(* Logix 5000 AddOnInstructionDefinition export Banner_S15C_UI_Param_v2; software revision 32.00 *)

TYPE Banner_IOL_Port_v2 :   // UDT that has all of the data items necessary to communicate with a specific Port on a IO-Link Master
STRUCT
   Port_Controlled : INT;   // Each bit represents a port on an IO-Link Master. Set to 1 to tell AOI to control that port.
   Port_Activate : INT;   // Each bit represents a port on an IO-Link Master. When ON that port will process any commands in queue.
   Port_Read : INT;   // Each bit represents a port on an IO-Link Master. Used to determine when device AOI has requested a Read command.
   Port_Write : INT;   // Each bit represents a port on an IO-Link Master. Used to determine when device AOI has requested a Write command.
   Port_RW_Complete : INT;   // Each bit represents a port on an IO-Link Master. Tells device AOI that Read or Write request has been completed.
   Port_Device_Read : INT;
   Data_Transfer : SINT[70];   // Array to transfer data from IO-Master to device AOIs.
END_STRUCT
END_TYPE

TYPE Banner_S15C_UI_RD_v2 :   // All of the read parameters for a S15C-IU unit.
STRUCT
   Master_Cycle_Time : INT;
   Min_Cycle_Time : INT;
   M_Sequence_Capability : INT;
   IO_Link_Version_ID : INT;
   Process_Data_Input_Length : INT;
   Process_Data_Output_Length : INT;
   Combined_Vendor_ID : DINT;   // IO-Link Vendor ID
   Vendor_ID1 : INT;
   Vendor_ID2 : INT;
   Combined_Device_ID : DINT;   // IO-Link Device ID
   Device_ID1 : INT;
   Device_ID2 : INT;
   Device_ID3 : INT;
   Serial_Number : STRING;
   Product_Name : STRING;
   All_Time_Run_Time : DINT;   // Current All Time Run Timer.
   Model_Type : SINT;   // 0 = Voltage, 1 = Current
   MDC_Lower_Limit : DINT;
   MDC_Upper_Limit : DINT;
   MDC_Unit : DINT;   // 1209 = A, 1240 = V
   MDC_Scale : DINT;   // 260 = microAmps, 253 = microVolts
END_STRUCT
END_TYPE

TYPE Banner_S15C_UI_v2 :   // All of the parameters for a S15C.
STRUCT
   Initial_Global_Read : BOOL;   // Determines if all of the IO-Link data has been read into the PLC yet
   Command : INT;   // Value placed in here will activate a read or write to a specifc IO-Link Index
   Read_Data : Banner_S15C_UI_RD_v2;   // Read Only Data
   Write_Data : Banner_S15C_UI_WD_v2;   // Write Data
   Archive : Banner_S15C_UI_WD_v2;   // Archive Data
   Reset : BOOL;   // Resets AOI. This will force a complete parameter read of the sensor.
END_STRUCT
END_TYPE

TYPE Banner_S15C_UI_WD_v2 :   // UDT that stores the Write Data for a S15C-IU unit.
STRUCT
   System_Command : INT;   // See IODD file for list of commands that can be activated via the System Command interface
   Parameter_Access_Lock : SINT;   // Write access to all parameters is prohibited while value is 1. Only this parameter can be adjusted when value is 1.
   Data_Storage_Lock : SINT;   // Automatic data storage is disabled when this value is equal to 1. Read access is not affected.
   Local_Parameterization_Lock : SINT;   // Parameterization via local control elements on device is disabled.
   Local_User_Interface_Lock : SINT;   // Operation of local user interface is disabled.
   Setpoint_SP1 : DINT;
   Setpoint_SP2 : DINT;
   Switchpoint_Logic : INT;   // 0 = Light Operate, 1 = Dark Operate
   BDC_Mode : INT;   // 2 = Window Mode.
   Hysteresis : DINT;   // Hysteresis value for the switchpoint.
   Resetable_Run_Time : DINT;   // Current Resetable Run Timer.
   PDI_Configuration : INT;   // 0 = Analog Value, 1 = Digital Measuring Sensor
   IOL_Filter_Time : DINT;   // Time to average IOL Process Data management between updates.
   All_Time_Run_Time_Event_Time : DINT;   // Time before an Event is generated. 0 = disable all-time event.
   Resetable_Run_Time_Event_Time : DINT;   // Time before an Event is generated. 0 = disable run time event.
END_STRUCT
END_TYPE

ADD_ON_INSTRUCTION Banner_S15C_UI_Param_v2   (* revision 2.1, vendor Banner Engineering *)
// AOI to read and write parameter data to an IO-Link S15C-I or S15C-U.
VAR_IN_OUT
   S15C : Banner_S15C_UI_v2; {required}
   Port_Data : Banner_IOL_Port_v2; {required}
END_VAR
VAR_INPUT
   Port : DINT; {required}
END_VAR
VAR
   Local_Control : DINT; {access None}
   Global_Read_Command_Value : INT; {access None}
   Global_Write_Command_Value : INT; {access None}
   Error_Generated : BOOL; {access None}
   Command_Being_Processed : BOOL; {access None}
   Index_Write_Inprocess : INT; {access None}
   Index_Write_Control : INT; {access None}
   Update_Archive : BOOL; {access None}
   Inprocess_Index : DINT; {access None}
END_VAR

ROUTINE Logic   (* ladder *)
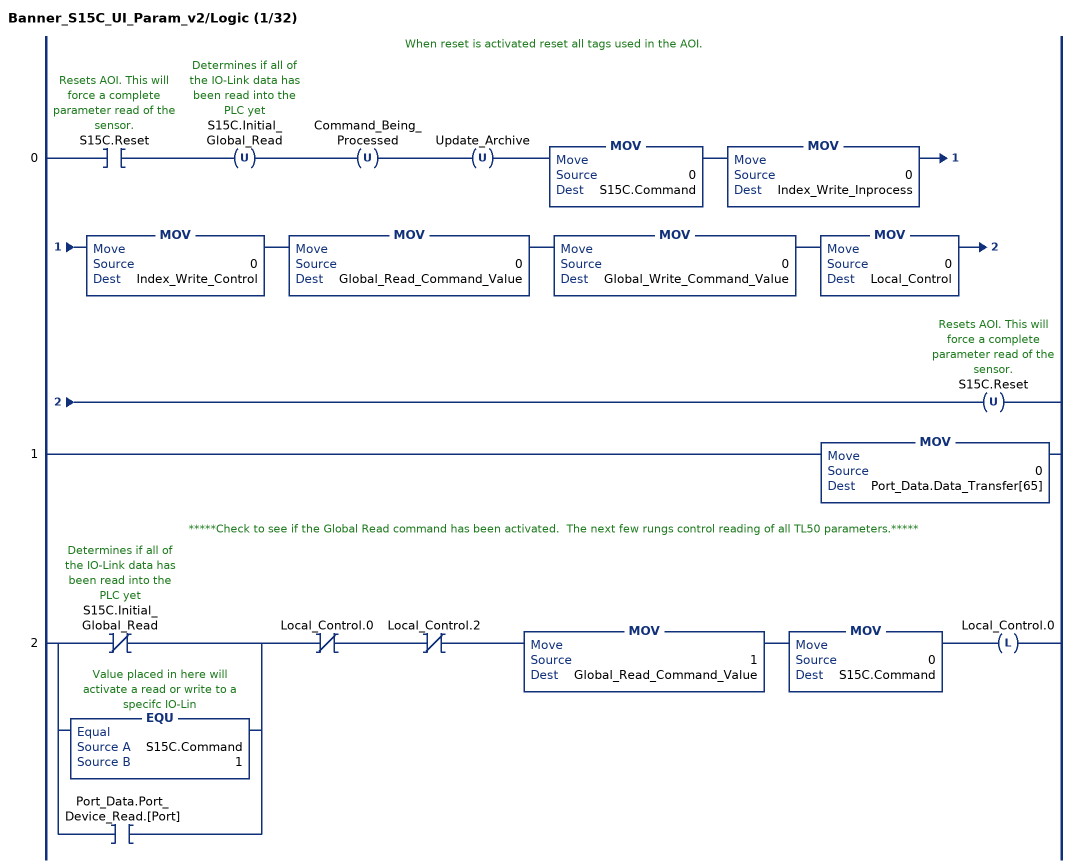
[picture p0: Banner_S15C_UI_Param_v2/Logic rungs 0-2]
   // When reset is activated reset all tags used in the AOI.
   0: XIC(S15C.Reset)OTU(S15C.Initial_Global_Read)OTU(Command_Being_Processed)OTU(Update_Archive)MOV(0,S15C.Command)MOV(0,Index_Write_Inprocess)MOV(0,Index_Write_Control)MOV(0,Global_Read_Command_Value)MOV(0,Global_Write_Command_Value)MOV(0,Local_Control)OTU(S15C.Reset);
   1: MOV(0,Port_Data.Data_Transfer[65]);
   // *****Check to see if the Global Read command has been activated.  The next few rungs control reading of all TL50 parameters.*****
   2: [XIO(S15C.Initial_Global_Read) ,EQU(S15C.Command,1) ,XIC(Port_Data.Port_Device_Read.[Port]) ]XIO(Local_Control.0)XIO(Local_Control.2)MOV(1,Global_Read_Command_Value)MOV(0,S15C.Command)OTL(Local_Control.0);
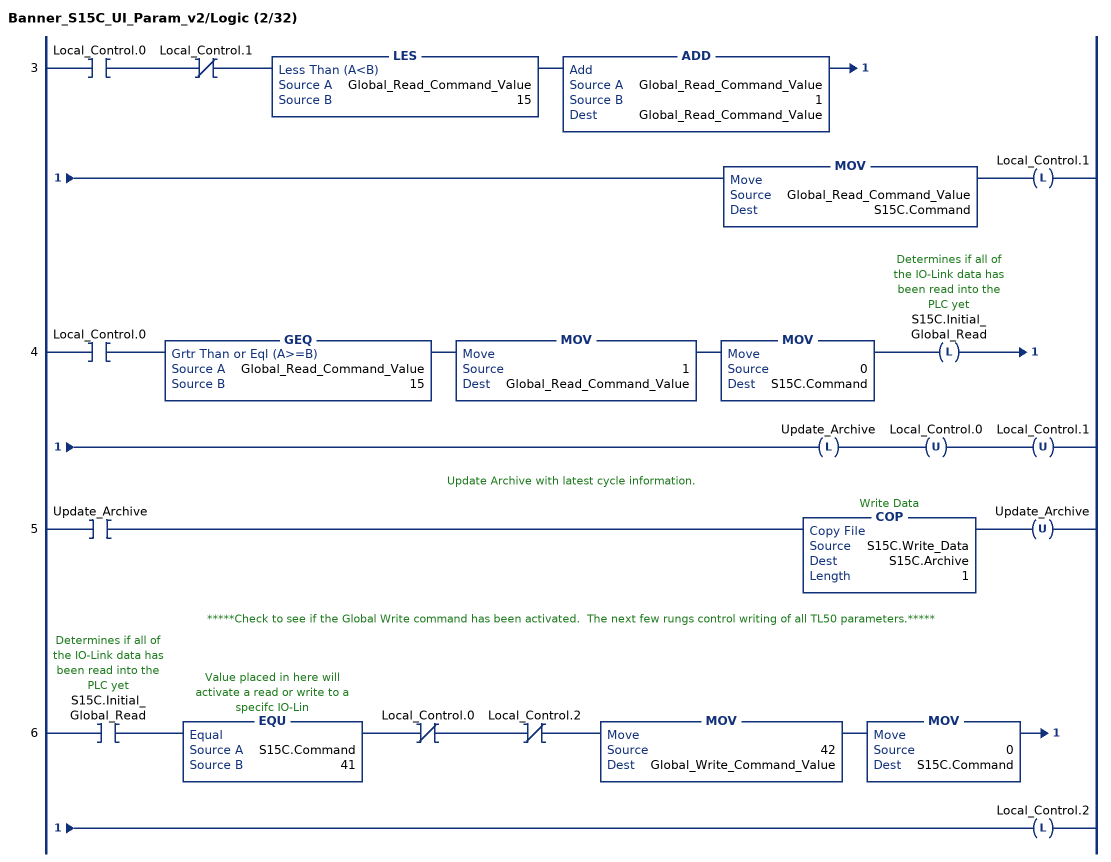
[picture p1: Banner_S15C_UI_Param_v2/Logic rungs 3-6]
   3: XIC(Local_Control.0)XIO(Local_Control.1)LES(Global_Read_Command_Value,15)ADD(Global_Read_Command_Value,1,Global_Read_Command_Value)MOV(Global_Read_Command_Value,S15C.Command)OTL(Local_Control.1);
   4: XIC(Local_Control.0)GEQ(Global_Read_Command_Value,15)MOV(1,Global_Read_Command_Value)MOV(0,S15C.Command)OTL(S15C.Initial_Global_Read)OTL(Update_Archive)OTU(Local_Control.0)OTU(Local_Control.1);
   // Update Archive with latest cycle information.
   5: XIC(Update_Archive)COP(S15C.Write_Data,S15C.Archive,1)OTU(Update_Archive);
   // *****Check to see if the Global Write command has been activated.  The next few rungs control writing of all TL50 parameters.*****
   6: XIC(S15C.Initial_Global_Read)EQU(S15C.Command,41)XIO(Local_Control.0)XIO(Local_Control.2)MOV(42,Global_Write_Command_Value)MOV(0,S15C.Command)OTL(Local_Control.2);
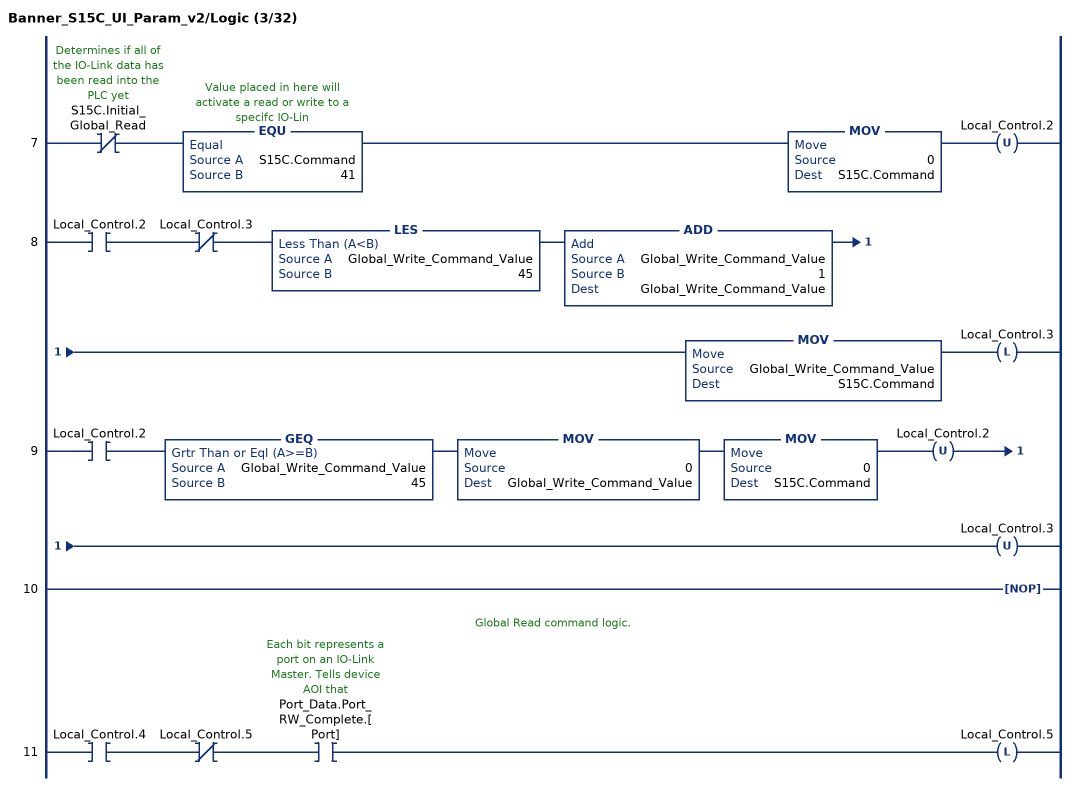
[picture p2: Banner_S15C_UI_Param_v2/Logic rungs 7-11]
   7: XIO(S15C.Initial_Global_Read)EQU(S15C.Command,41)MOV(0,S15C.Command)OTU(Local_Control.2);
   8: XIC(Local_Control.2)XIO(Local_Control.3)LES(Global_Write_Command_Value,45)ADD(Global_Write_Command_Value,1,Global_Write_Command_Value)MOV(Global_Write_Command_Value,S15C.Command)OTL(Local_Control.3);
   9: XIC(Local_Control.2)GEQ(Global_Write_Command_Value,45)MOV(0,Global_Write_Command_Value)MOV(0,S15C.Command)OTU(Local_Control.2)OTU(Local_Control.3);
   10: NOP();
   // Global Read command logic.
   11: XIC(Local_Control.4)XIO(Local_Control.5)XIC(Port_Data.Port_RW_Complete.[Port])OTL(Local_Control.5);
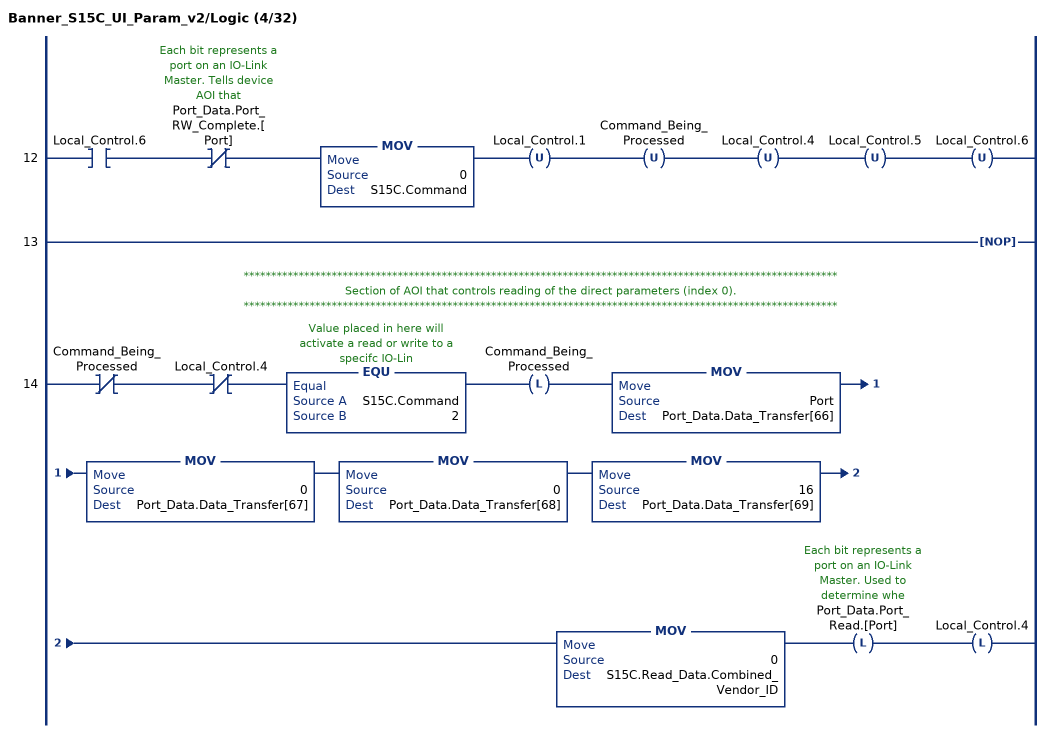
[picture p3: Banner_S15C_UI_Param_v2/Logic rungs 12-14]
   12: XIC(Local_Control.6)XIO(Port_Data.Port_RW_Complete.[Port])MOV(0,S15C.Command)OTU(Local_Control.1)OTU(Command_Being_Processed)OTU(Local_Control.4)OTU(Local_Control.5)OTU(Local_Control.6);
   13: NOP();
   // ************************************************************************************************************
   // Section of AOI that controls reading of the direct parameters (index 0).
   // ************************************************************************************************************
   14: XIO(Command_Being_Processed)XIO(Local_Control.4)EQU(S15C.Command,2)OTL(Command_Being_Processed)MOV(Port,Port_Data.Data_Transfer[66])MOV(0,Port_Data.Data_Transfer[67])MOV(0,Port_Data.Data_Transfer[68])MOV(16,Port_Data.Data_Transfer[69])MOV(0,S15C.Read_Data.Combined_Vendor_ID)OTL(Port_Data.Port_Read.[Port])OTL(Local_Control.4);
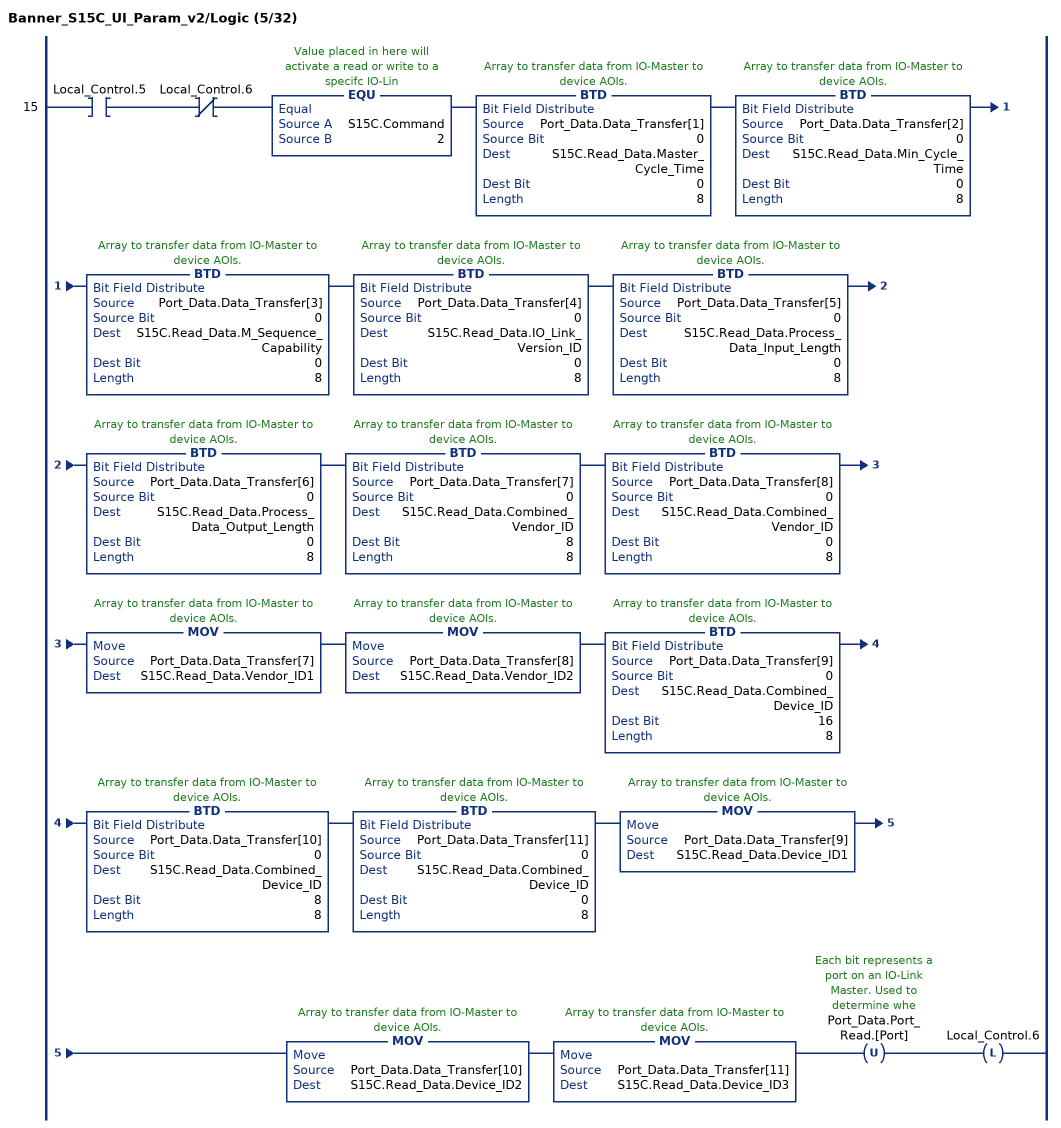
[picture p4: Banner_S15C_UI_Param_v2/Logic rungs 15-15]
   15: XIC(Local_Control.5)XIO(Local_Control.6)EQU(S15C.Command,2)BTD(Port_Data.Data_Transfer[1],0,S15C.Read_Data.Master_Cycle_Time,0,8)BTD(Port_Data.Data_Transfer[2],0,S15C.Read_Data.Min_Cycle_Time,0,8)BTD(Port_Data.Data_Transfer[3],0,S15C.Read_Data.M_Sequence_Capability,0,8)BTD(Port_Data.Data_Transfer[4],0,S15C.Read_Data.IO_Link_Version_ID,0,8)BTD(Port_Data.Data_Transfer[5],0,S15C.Read_Data.Process_Data_Input_Length,0,8)BTD(Port_Data.Data_Transfer[6],0,S15C.Read_Data.Process_Data_Output_Length,0,8)BTD(Port_Data.Data_Transfer[7],0,S15C.Read_Data.Combined_Vendor_ID,8,8)BTD(Port_Data.Data_Transfer[8],0,S15C.Read_Data.Combined_Vendor_ID,0,8)MOV(Port_Data.Data_Transfer[7],S15C.Read_Data.Vendor_ID1)MOV(Port_Data.Data_Transfer[8],S15C.Read_Data.Vendor_ID2)BTD(Port_Data.Data_Transfer[9],0,S15C.Read_Data.Combined_Device_ID,16,8)BTD(Port_Data.Data_Transfer[10],0,S15C.Read_Data.Combined_Device_ID,8,8)BTD(Port_Data.Data_Transfer[11],0,S15C.Read_Data.Combined_Device_ID,0,8)MOV(Port_Data.Data_Transfer[9],S15C.Read_Data.Device_ID1)MOV(Port_Data.Data_Transfer[10],S15C.Read_Data.Device_ID2)MOV(Port_Data.Data_Transfer[11],S15C.Read_Data.Device_ID3)OTU(Port_Data.Port_Read.[Port])OTL(Local_Control.6);
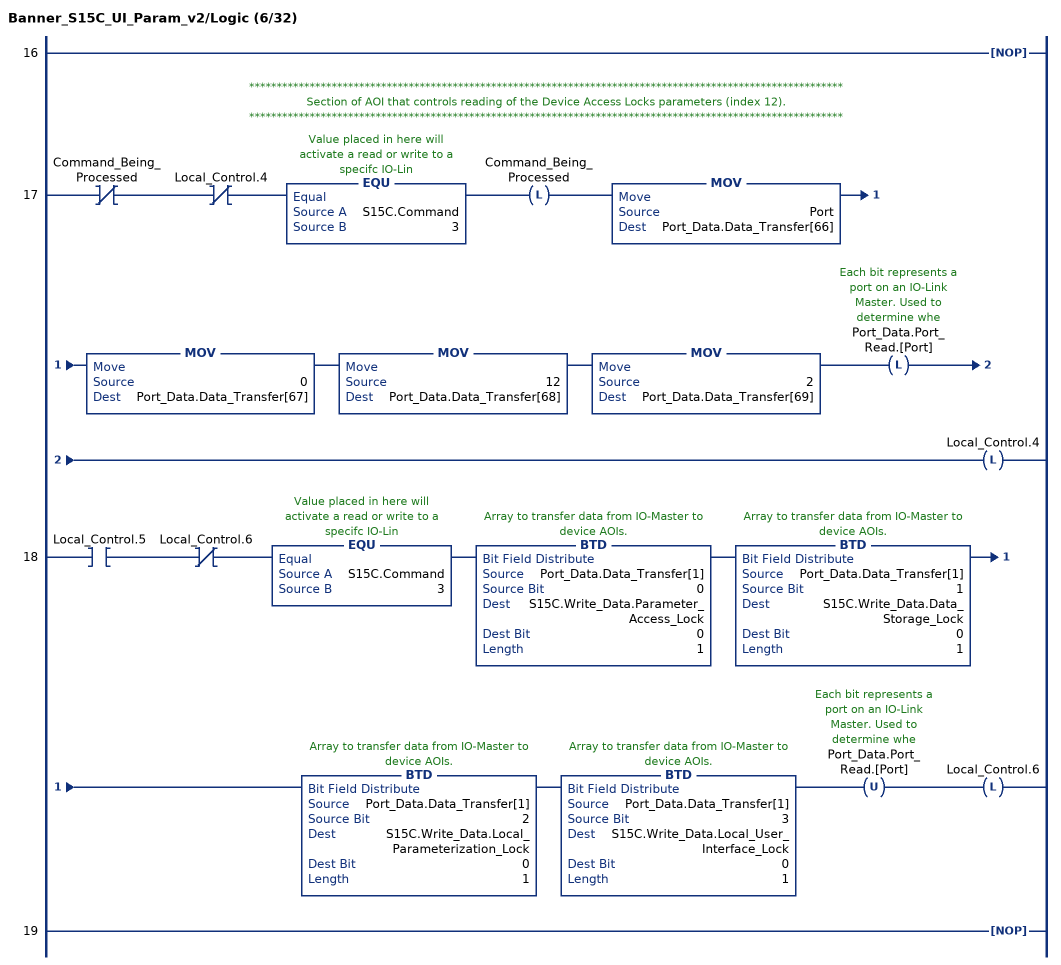
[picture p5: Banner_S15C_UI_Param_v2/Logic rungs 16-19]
   16: NOP();
   // ************************************************************************************************************
   // Section of AOI that controls reading of the Device Access Locks parameters (index 12).
   // ************************************************************************************************************
   17: XIO(Command_Being_Processed)XIO(Local_Control.4)EQU(S15C.Command,3)OTL(Command_Being_Processed)MOV(Port,Port_Data.Data_Transfer[66])MOV(0,Port_Data.Data_Transfer[67])MOV(12,Port_Data.Data_Transfer[68])MOV(2,Port_Data.Data_Transfer[69])OTL(Port_Data.Port_Read.[Port])OTL(Local_Control.4);
   18: XIC(Local_Control.5)XIO(Local_Control.6)EQU(S15C.Command,3)BTD(Port_Data.Data_Transfer[1],0,S15C.Write_Data.Parameter_Access_Lock,0,1)BTD(Port_Data.Data_Transfer[1],1,S15C.Write_Data.Data_Storage_Lock,0,1)BTD(Port_Data.Data_Transfer[1],2,S15C.Write_Data.Local_Parameterization_Lock,0,1)BTD(Port_Data.Data_Transfer[1],3,S15C.Write_Data.Local_User_Interface_Lock,0,1)OTU(Port_Data.Port_Read.[Port])OTL(Local_Control.6);
   19: NOP();
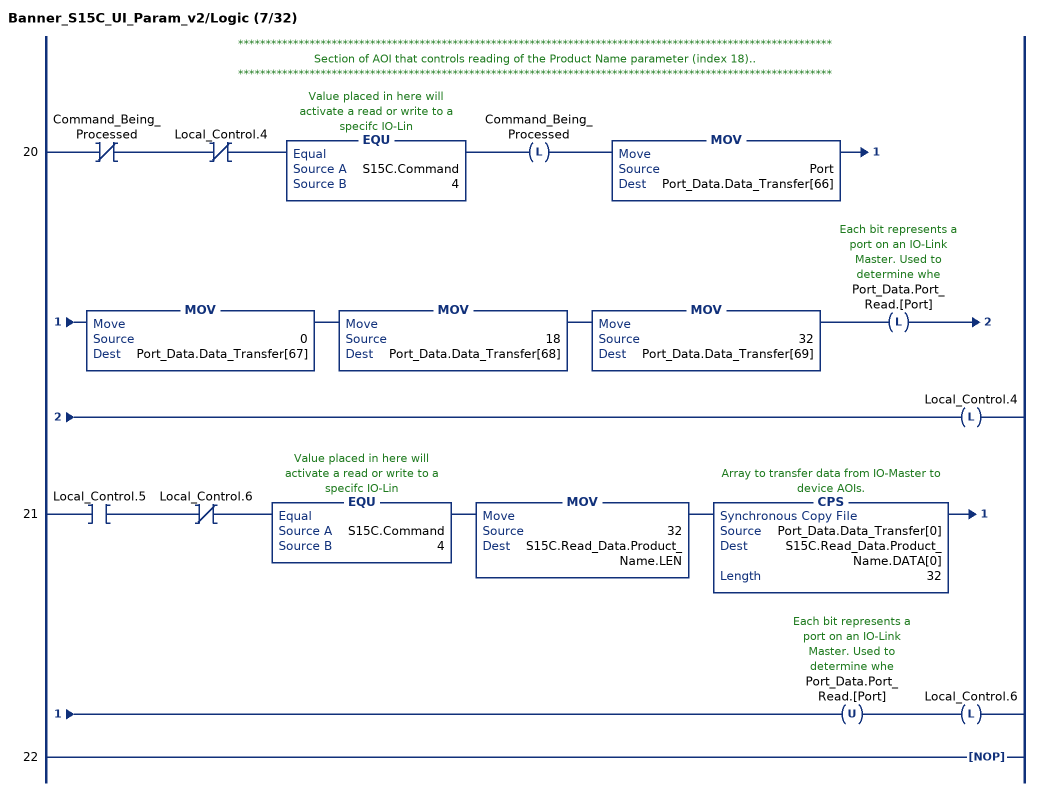
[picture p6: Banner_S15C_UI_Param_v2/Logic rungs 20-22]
   // ************************************************************************************************************
   // Section of AOI that controls reading of the Product Name parameter (index 18)..
   // ************************************************************************************************************
   20: XIO(Command_Being_Processed)XIO(Local_Control.4)EQU(S15C.Command,4)OTL(Command_Being_Processed)MOV(Port,Port_Data.Data_Transfer[66])MOV(0,Port_Data.Data_Transfer[67])MOV(18,Port_Data.Data_Transfer[68])MOV(32,Port_Data.Data_Transfer[69])OTL(Port_Data.Port_Read.[Port])OTL(Local_Control.4);
   21: XIC(Local_Control.5)XIO(Local_Control.6)EQU(S15C.Command,4)MOV(32,S15C.Read_Data.Product_Name.LEN)CPS(Port_Data.Data_Transfer[0],S15C.Read_Data.Product_Name.DATA[0],32)OTU(Port_Data.Port_Read.[Port])OTL(Local_Control.6);
   22: NOP();
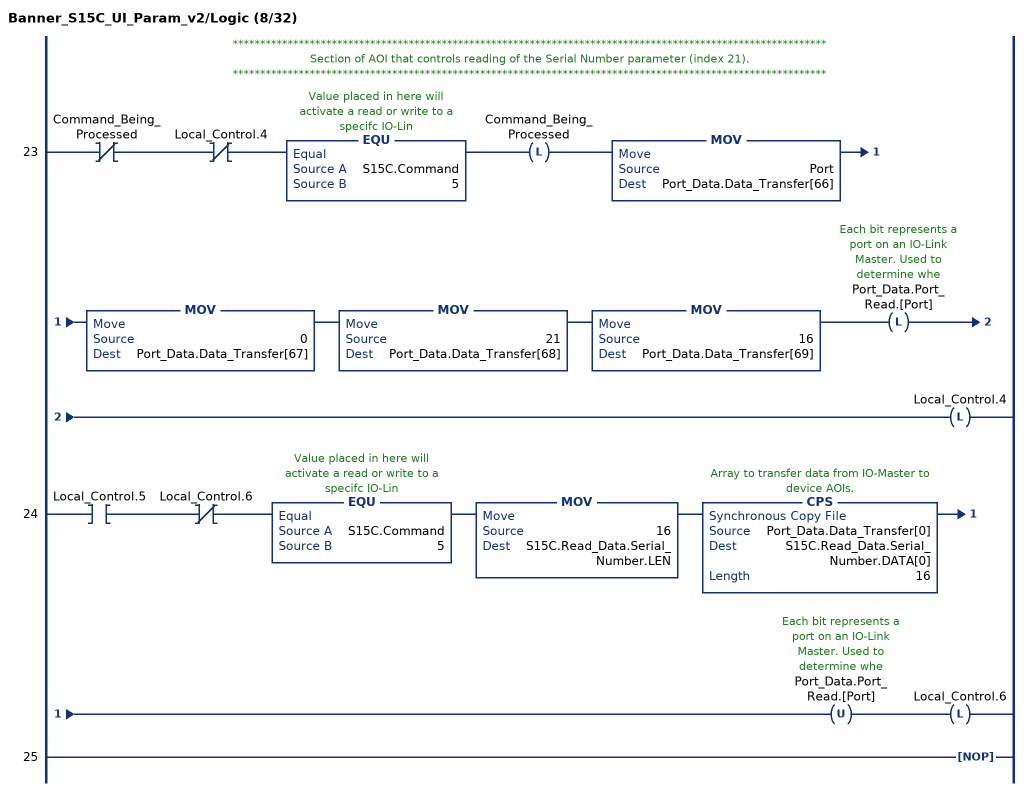
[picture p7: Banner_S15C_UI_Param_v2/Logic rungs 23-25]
   // ************************************************************************************************************
   // Section of AOI that controls reading of the Serial Number parameter (index 21).
   // ************************************************************************************************************
   23: XIO(Command_Being_Processed)XIO(Local_Control.4)EQU(S15C.Command,5)OTL(Command_Being_Processed)MOV(Port,Port_Data.Data_Transfer[66])MOV(0,Port_Data.Data_Transfer[67])MOV(21,Port_Data.Data_Transfer[68])MOV(16,Port_Data.Data_Transfer[69])OTL(Port_Data.Port_Read.[Port])OTL(Local_Control.4);
   24: XIC(Local_Control.5)XIO(Local_Control.6)EQU(S15C.Command,5)MOV(16,S15C.Read_Data.Serial_Number.LEN)CPS(Port_Data.Data_Transfer[0],S15C.Read_Data.Serial_Number.DATA[0],16)OTU(Port_Data.Port_Read.[Port])OTL(Local_Control.6);
   25: NOP();
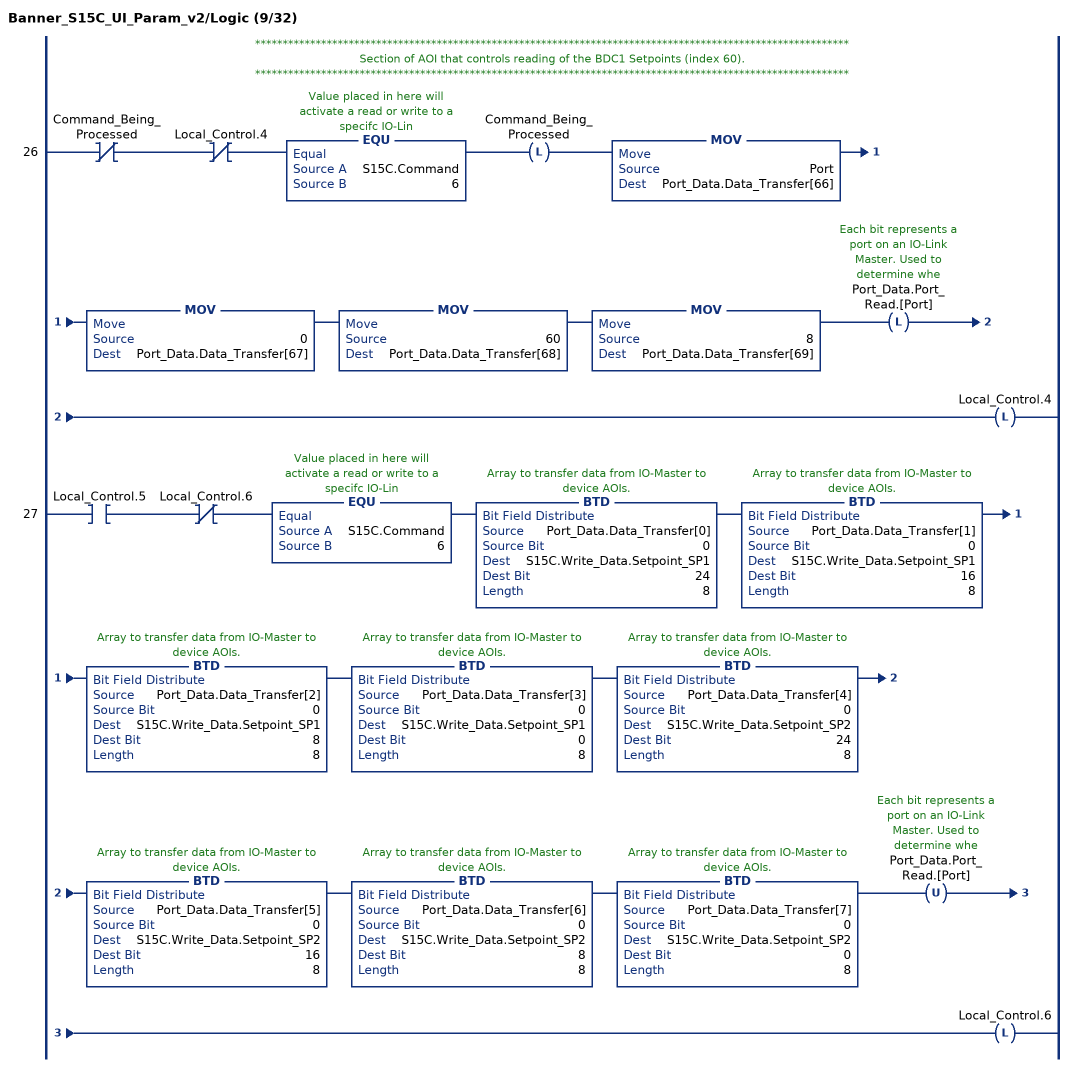
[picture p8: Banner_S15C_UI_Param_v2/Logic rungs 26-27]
   // ************************************************************************************************************
   // Section of AOI that controls reading of the BDC1 Setpoints (index 60).
   // ************************************************************************************************************
   26: XIO(Command_Being_Processed)XIO(Local_Control.4)EQU(S15C.Command,6)OTL(Command_Being_Processed)MOV(Port,Port_Data.Data_Transfer[66])MOV(0,Port_Data.Data_Transfer[67])MOV(60,Port_Data.Data_Transfer[68])MOV(8,Port_Data.Data_Transfer[69])OTL(Port_Data.Port_Read.[Port])OTL(Local_Control.4);
   27: XIC(Local_Control.5)XIO(Local_Control.6)EQU(S15C.Command,6)BTD(Port_Data.Data_Transfer[0],0,S15C.Write_Data.Setpoint_SP1,24,8)BTD(Port_Data.Data_Transfer[1],0,S15C.Write_Data.Setpoint_SP1,16,8)BTD(Port_Data.Data_Transfer[2],0,S15C.Write_Data.Setpoint_SP1,8,8)BTD(Port_Data.Data_Transfer[3],0,S15C.Write_Data.Setpoint_SP1,0,8)BTD(Port_Data.Data_Transfer[4],0,S15C.Write_Data.Setpoint_SP2,24,8)BTD(Port_Data.Data_Transfer[5],0,S15C.Write_Data.Setpoint_SP2,16,8)BTD(Port_Data.Data_Transfer[6],0,S15C.Write_Data.Setpoint_SP2,8,8)BTD(Port_Data.Data_Transfer[7],0,S15C.Write_Data.Setpoint_SP2,0,8)OTU(Port_Data.Port_Read.[Port])OTL(Local_Control.6);
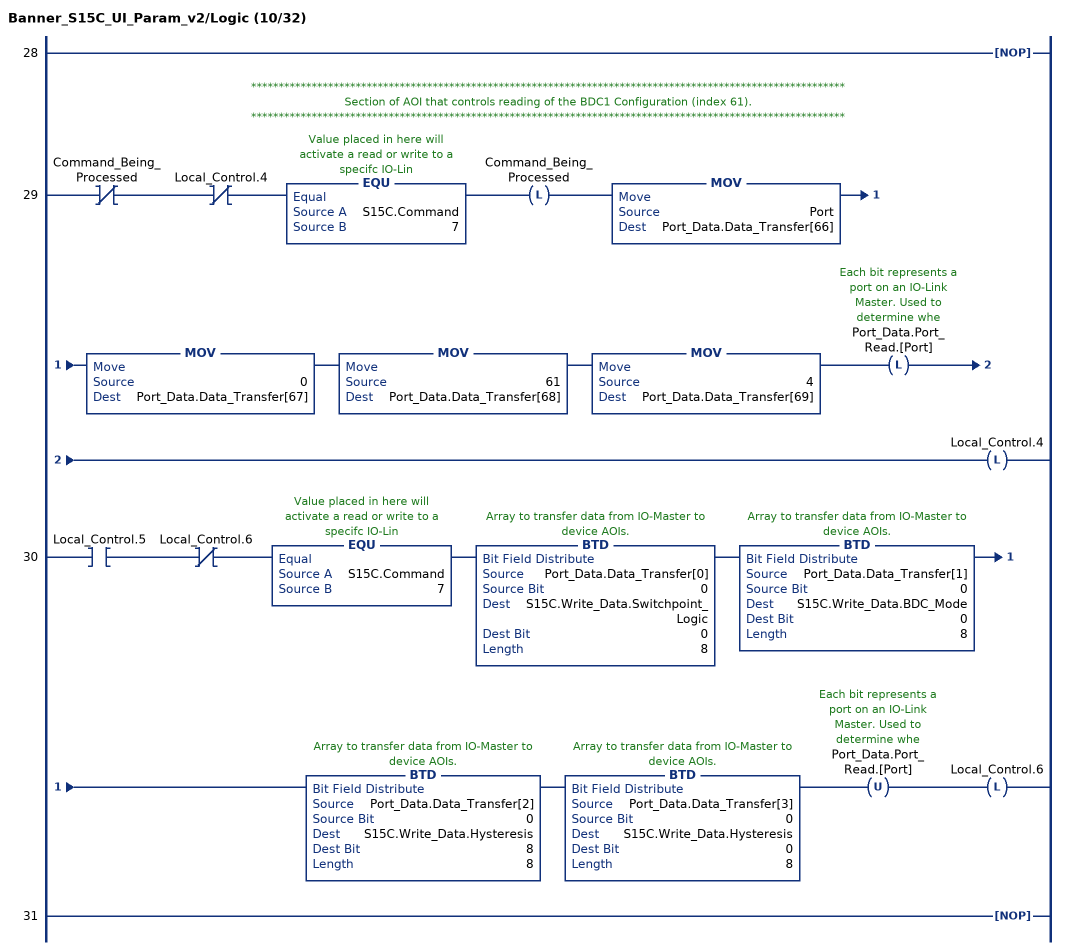
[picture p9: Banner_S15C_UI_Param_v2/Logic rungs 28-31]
   28: NOP();
   // ************************************************************************************************************
   // Section of AOI that controls reading of the BDC1 Configuration (index 61).
   // ************************************************************************************************************
   29: XIO(Command_Being_Processed)XIO(Local_Control.4)EQU(S15C.Command,7)OTL(Command_Being_Processed)MOV(Port,Port_Data.Data_Transfer[66])MOV(0,Port_Data.Data_Transfer[67])MOV(61,Port_Data.Data_Transfer[68])MOV(4,Port_Data.Data_Transfer[69])OTL(Port_Data.Port_Read.[Port])OTL(Local_Control.4);
   30: XIC(Local_Control.5)XIO(Local_Control.6)EQU(S15C.Command,7)BTD(Port_Data.Data_Transfer[0],0,S15C.Write_Data.Switchpoint_Logic,0,8)BTD(Port_Data.Data_Transfer[1],0,S15C.Write_Data.BDC_Mode,0,8)BTD(Port_Data.Data_Transfer[2],0,S15C.Write_Data.Hysteresis,8,8)BTD(Port_Data.Data_Transfer[3],0,S15C.Write_Data.Hysteresis,0,8)OTU(Port_Data.Port_Read.[Port])OTL(Local_Control.6);
   31: NOP();
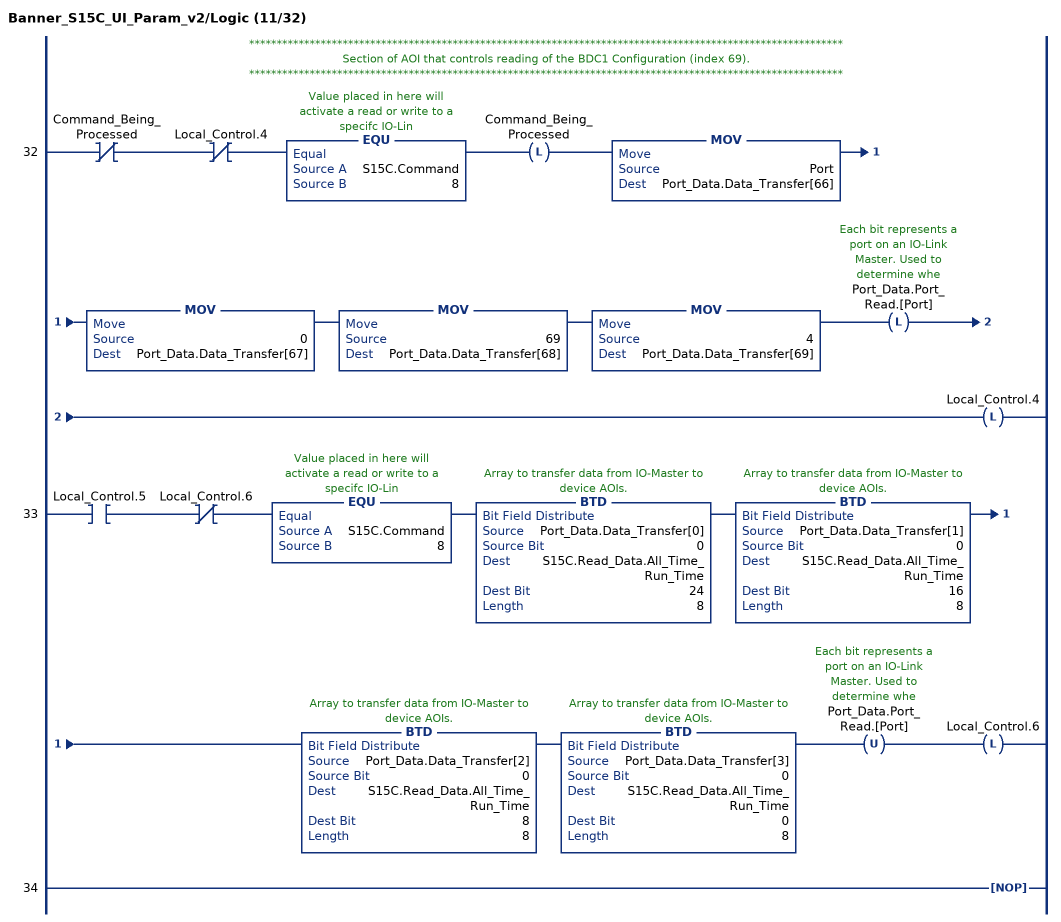
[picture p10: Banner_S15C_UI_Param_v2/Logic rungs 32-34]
   // ************************************************************************************************************
   // Section of AOI that controls reading of the BDC1 Configuration (index 69).
   // ************************************************************************************************************
   32: XIO(Command_Being_Processed)XIO(Local_Control.4)EQU(S15C.Command,8)OTL(Command_Being_Processed)MOV(Port,Port_Data.Data_Transfer[66])MOV(0,Port_Data.Data_Transfer[67])MOV(69,Port_Data.Data_Transfer[68])MOV(4,Port_Data.Data_Transfer[69])OTL(Port_Data.Port_Read.[Port])OTL(Local_Control.4);
   33: XIC(Local_Control.5)XIO(Local_Control.6)EQU(S15C.Command,8)BTD(Port_Data.Data_Transfer[0],0,S15C.Read_Data.All_Time_Run_Time,24,8)BTD(Port_Data.Data_Transfer[1],0,S15C.Read_Data.All_Time_Run_Time,16,8)BTD(Port_Data.Data_Transfer[2],0,S15C.Read_Data.All_Time_Run_Time,8,8)BTD(Port_Data.Data_Transfer[3],0,S15C.Read_Data.All_Time_Run_Time,0,8)OTU(Port_Data.Port_Read.[Port])OTL(Local_Control.6);
   34: NOP();
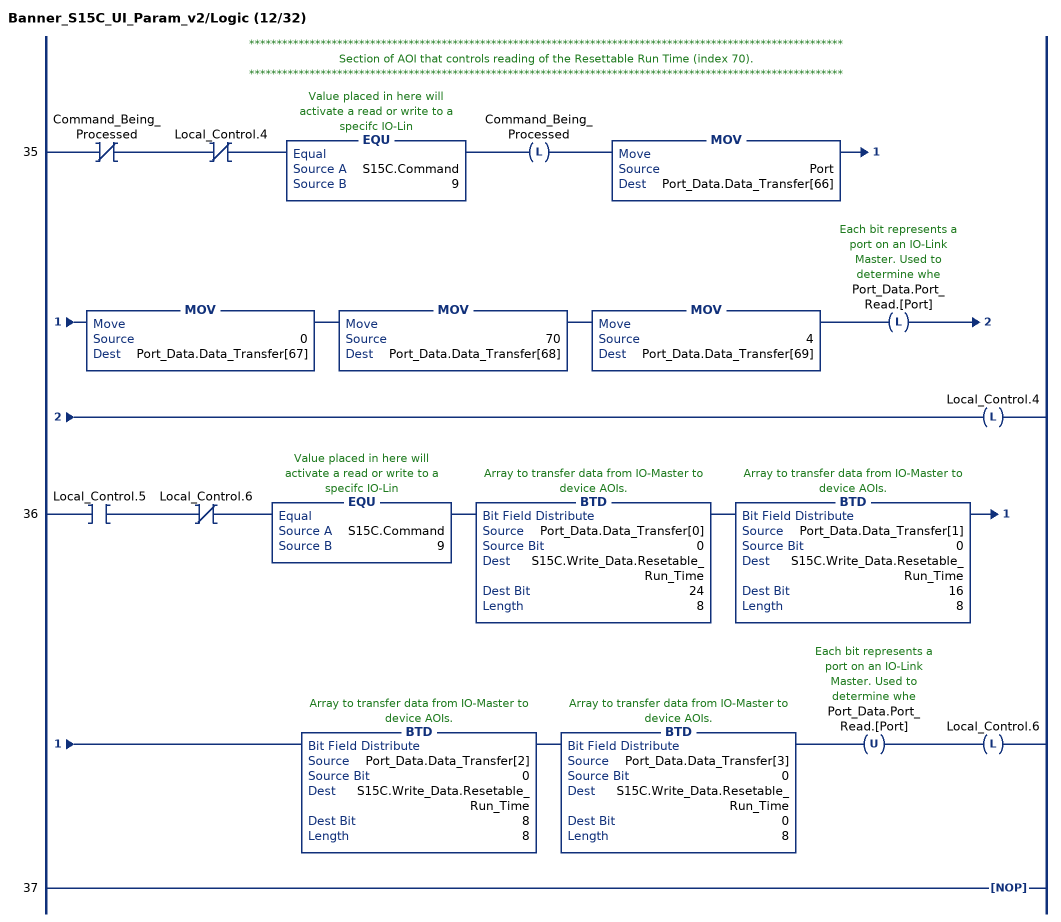
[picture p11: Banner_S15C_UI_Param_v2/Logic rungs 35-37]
   // ************************************************************************************************************
   // Section of AOI that controls reading of the Resettable Run Time (index 70).
   // ************************************************************************************************************
   35: XIO(Command_Being_Processed)XIO(Local_Control.4)EQU(S15C.Command,9)OTL(Command_Being_Processed)MOV(Port,Port_Data.Data_Transfer[66])MOV(0,Port_Data.Data_Transfer[67])MOV(70,Port_Data.Data_Transfer[68])MOV(4,Port_Data.Data_Transfer[69])OTL(Port_Data.Port_Read.[Port])OTL(Local_Control.4);
   36: XIC(Local_Control.5)XIO(Local_Control.6)EQU(S15C.Command,9)BTD(Port_Data.Data_Transfer[0],0,S15C.Write_Data.Resetable_Run_Time,24,8)BTD(Port_Data.Data_Transfer[1],0,S15C.Write_Data.Resetable_Run_Time,16,8)BTD(Port_Data.Data_Transfer[2],0,S15C.Write_Data.Resetable_Run_Time,8,8)BTD(Port_Data.Data_Transfer[3],0,S15C.Write_Data.Resetable_Run_Time,0,8)OTU(Port_Data.Port_Read.[Port])OTL(Local_Control.6);
   37: NOP();
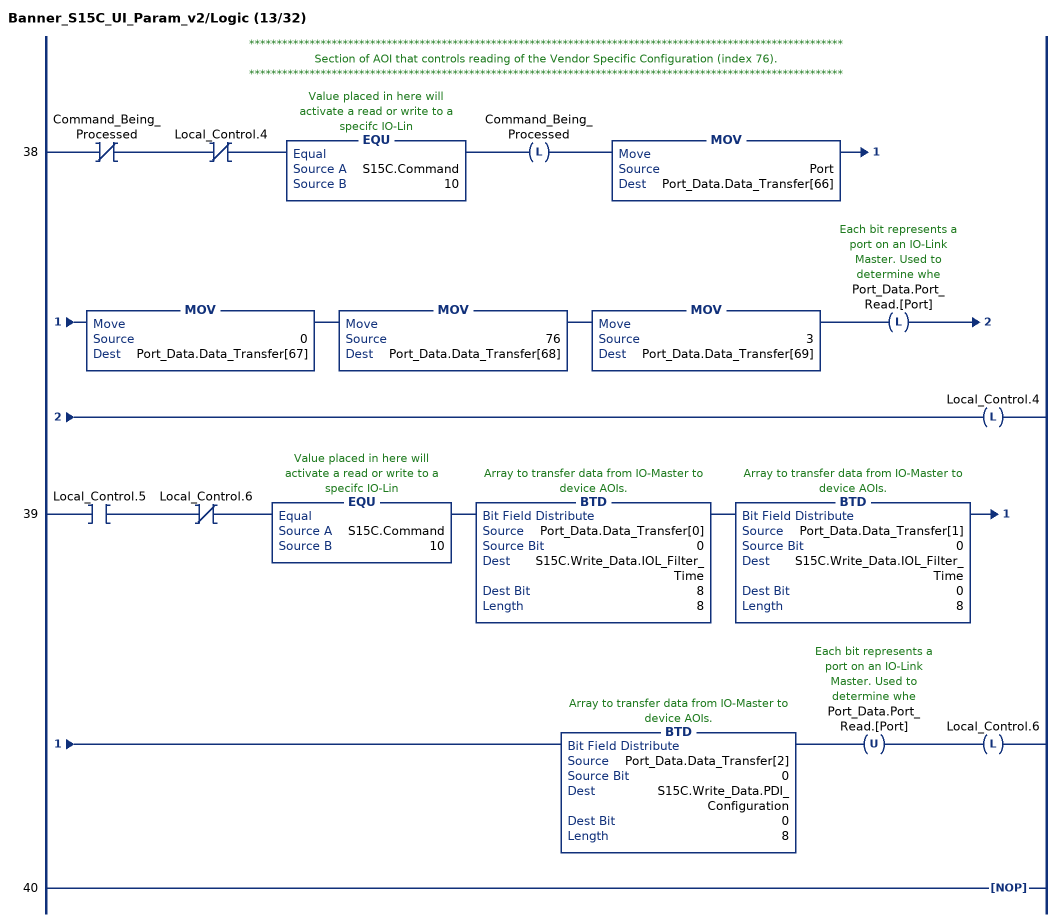
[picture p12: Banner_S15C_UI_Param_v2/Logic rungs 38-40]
   // ************************************************************************************************************
   // Section of AOI that controls reading of the Vendor Specific Configuration (index 76).
   // ************************************************************************************************************
   38: XIO(Command_Being_Processed)XIO(Local_Control.4)EQU(S15C.Command,10)OTL(Command_Being_Processed)MOV(Port,Port_Data.Data_Transfer[66])MOV(0,Port_Data.Data_Transfer[67])MOV(76,Port_Data.Data_Transfer[68])MOV(3,Port_Data.Data_Transfer[69])OTL(Port_Data.Port_Read.[Port])OTL(Local_Control.4);
   39: XIC(Local_Control.5)XIO(Local_Control.6)EQU(S15C.Command,10)BTD(Port_Data.Data_Transfer[0],0,S15C.Write_Data.IOL_Filter_Time,8,8)BTD(Port_Data.Data_Transfer[1],0,S15C.Write_Data.IOL_Filter_Time,0,8)BTD(Port_Data.Data_Transfer[2],0,S15C.Write_Data.PDI_Configuration,0,8)OTU(Port_Data.Port_Read.[Port])OTL(Local_Control.6);
   40: NOP();
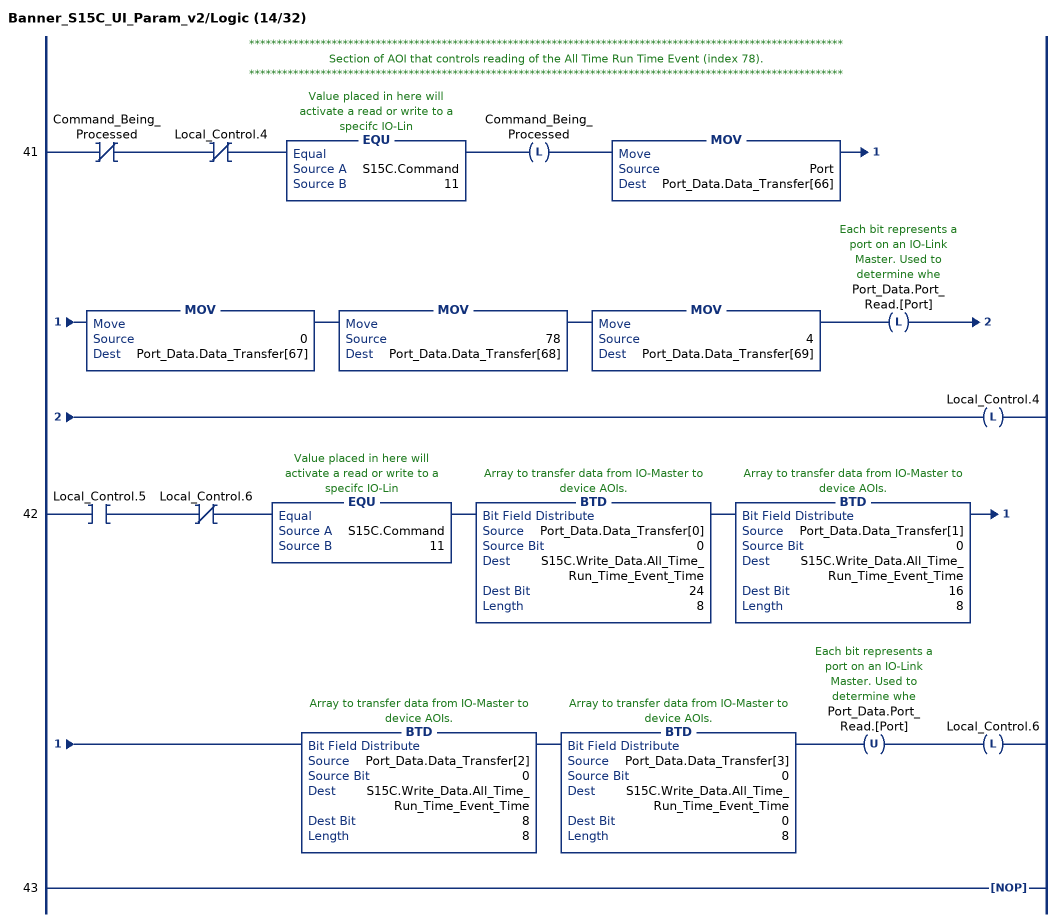
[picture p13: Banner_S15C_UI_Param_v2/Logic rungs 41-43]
   // ************************************************************************************************************
   // Section of AOI that controls reading of the All Time Run Time Event (index 78).
   // ************************************************************************************************************
   41: XIO(Command_Being_Processed)XIO(Local_Control.4)EQU(S15C.Command,11)OTL(Command_Being_Processed)MOV(Port,Port_Data.Data_Transfer[66])MOV(0,Port_Data.Data_Transfer[67])MOV(78,Port_Data.Data_Transfer[68])MOV(4,Port_Data.Data_Transfer[69])OTL(Port_Data.Port_Read.[Port])OTL(Local_Control.4);
   42: XIC(Local_Control.5)XIO(Local_Control.6)EQU(S15C.Command,11)BTD(Port_Data.Data_Transfer[0],0,S15C.Write_Data.All_Time_Run_Time_Event_Time,24,8)BTD(Port_Data.Data_Transfer[1],0,S15C.Write_Data.All_Time_Run_Time_Event_Time,16,8)BTD(Port_Data.Data_Transfer[2],0,S15C.Write_Data.All_Time_Run_Time_Event_Time,8,8)BTD(Port_Data.Data_Transfer[3],0,S15C.Write_Data.All_Time_Run_Time_Event_Time,0,8)OTU(Port_Data.Port_Read.[Port])OTL(Local_Control.6);
   43: NOP();
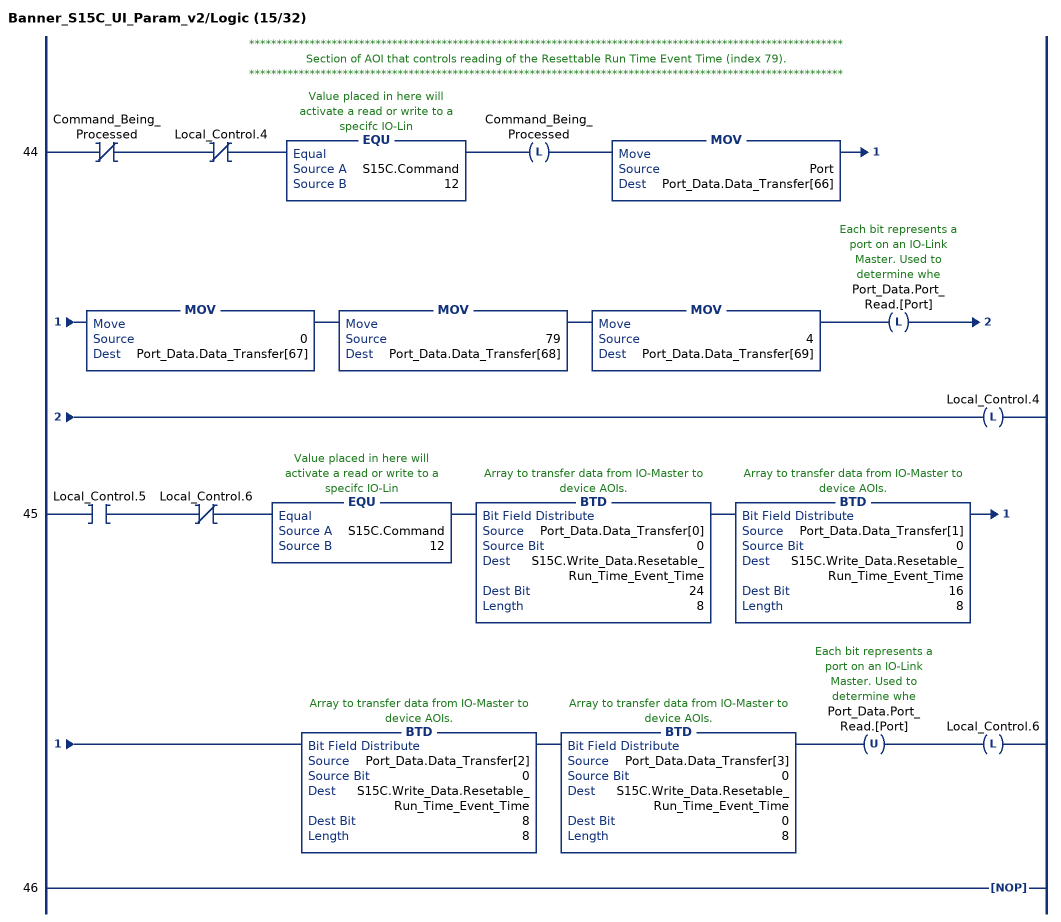
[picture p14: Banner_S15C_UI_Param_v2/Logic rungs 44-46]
   // ************************************************************************************************************
   // Section of AOI that controls reading of the Resettable Run Time Event Time (index 79).
   // ************************************************************************************************************
   44: XIO(Command_Being_Processed)XIO(Local_Control.4)EQU(S15C.Command,12)OTL(Command_Being_Processed)MOV(Port,Port_Data.Data_Transfer[66])MOV(0,Port_Data.Data_Transfer[67])MOV(79,Port_Data.Data_Transfer[68])MOV(4,Port_Data.Data_Transfer[69])OTL(Port_Data.Port_Read.[Port])OTL(Local_Control.4);
   45: XIC(Local_Control.5)XIO(Local_Control.6)EQU(S15C.Command,12)BTD(Port_Data.Data_Transfer[0],0,S15C.Write_Data.Resetable_Run_Time_Event_Time,24,8)BTD(Port_Data.Data_Transfer[1],0,S15C.Write_Data.Resetable_Run_Time_Event_Time,16,8)BTD(Port_Data.Data_Transfer[2],0,S15C.Write_Data.Resetable_Run_Time_Event_Time,8,8)BTD(Port_Data.Data_Transfer[3],0,S15C.Write_Data.Resetable_Run_Time_Event_Time,0,8)OTU(Port_Data.Port_Read.[Port])OTL(Local_Control.6);
   46: NOP();
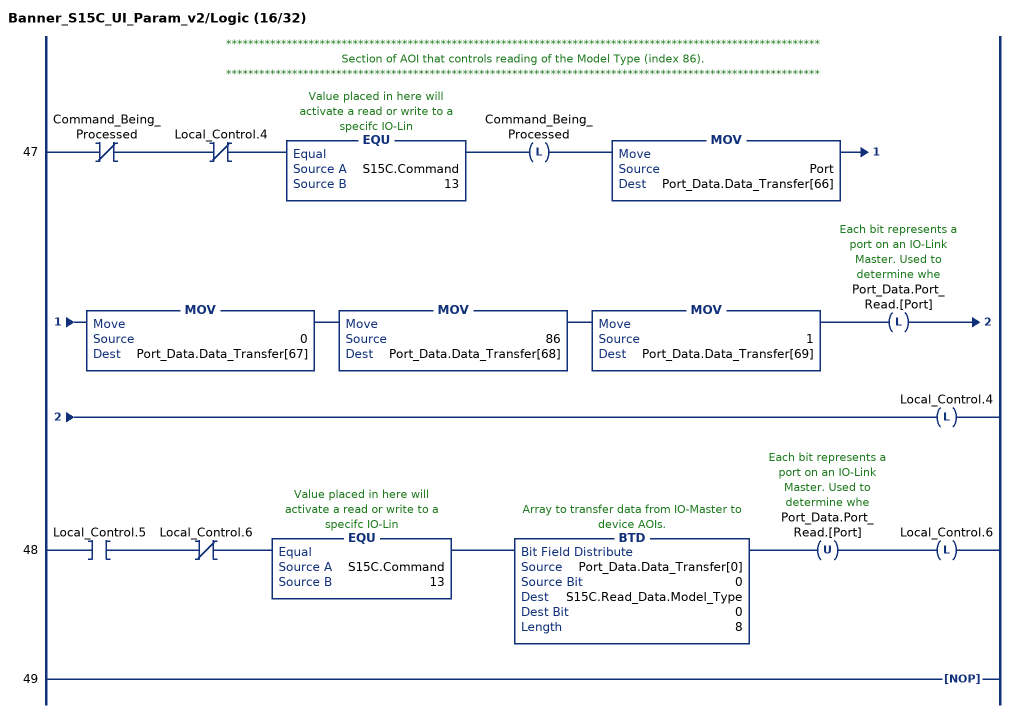
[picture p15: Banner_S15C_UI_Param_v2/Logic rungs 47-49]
   // ************************************************************************************************************
   // Section of AOI that controls reading of the Model Type (index 86).
   // ************************************************************************************************************
   47: XIO(Command_Being_Processed)XIO(Local_Control.4)EQU(S15C.Command,13)OTL(Command_Being_Processed)MOV(Port,Port_Data.Data_Transfer[66])MOV(0,Port_Data.Data_Transfer[67])MOV(86,Port_Data.Data_Transfer[68])MOV(1,Port_Data.Data_Transfer[69])OTL(Port_Data.Port_Read.[Port])OTL(Local_Control.4);
   48: XIC(Local_Control.5)XIO(Local_Control.6)EQU(S15C.Command,13)BTD(Port_Data.Data_Transfer[0],0,S15C.Read_Data.Model_Type,0,8)OTU(Port_Data.Port_Read.[Port])OTL(Local_Control.6);
   49: NOP();
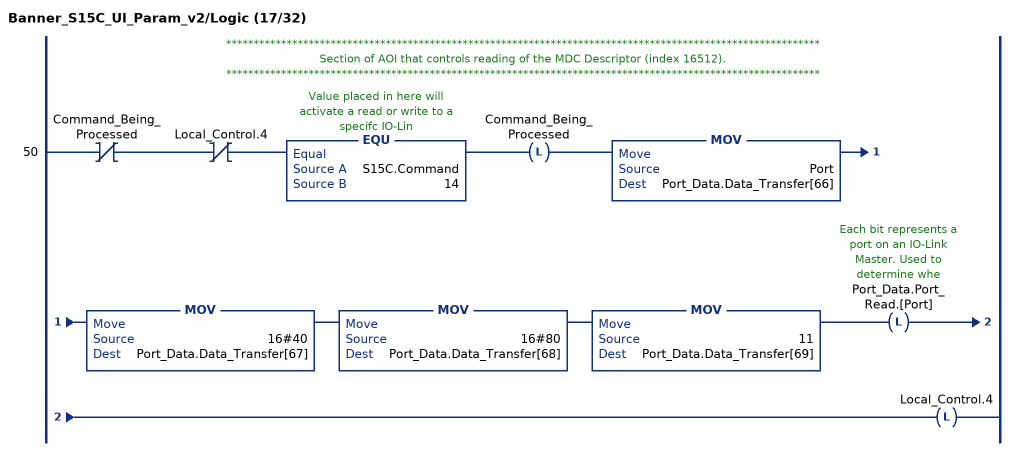
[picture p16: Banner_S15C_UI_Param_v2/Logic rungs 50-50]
   // ************************************************************************************************************
   // Section of AOI that controls reading of the MDC Descriptor (index 16512).
   // ************************************************************************************************************
   50: XIO(Command_Being_Processed)XIO(Local_Control.4)EQU(S15C.Command,14)OTL(Command_Being_Processed)MOV(Port,Port_Data.Data_Transfer[66])MOV(16#40,Port_Data.Data_Transfer[67])MOV(16#80,Port_Data.Data_Transfer[68])MOV(11,Port_Data.Data_Transfer[69])OTL(Port_Data.Port_Read.[Port])OTL(Local_Control.4);
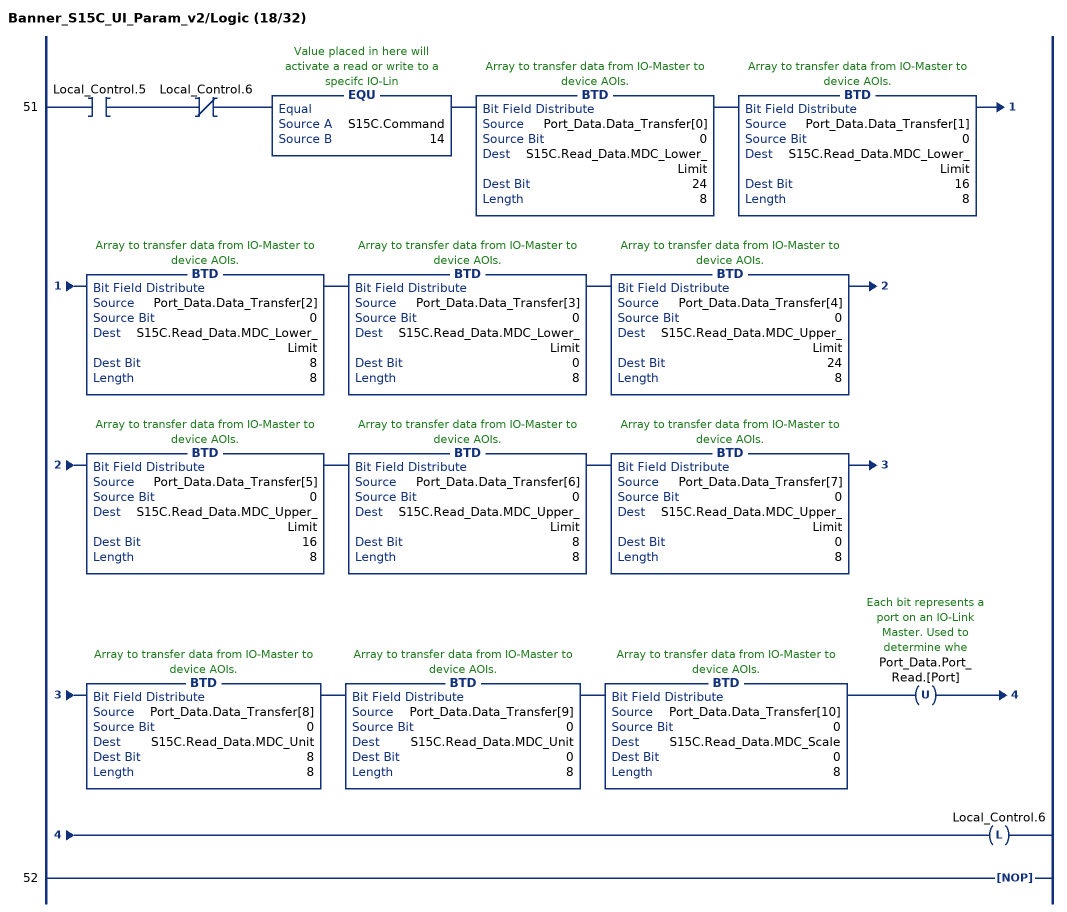
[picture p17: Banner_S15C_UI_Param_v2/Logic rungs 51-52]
   51: XIC(Local_Control.5)XIO(Local_Control.6)EQU(S15C.Command,14)BTD(Port_Data.Data_Transfer[0],0,S15C.Read_Data.MDC_Lower_Limit,24,8)BTD(Port_Data.Data_Transfer[1],0,S15C.Read_Data.MDC_Lower_Limit,16,8)BTD(Port_Data.Data_Transfer[2],0,S15C.Read_Data.MDC_Lower_Limit,8,8)BTD(Port_Data.Data_Transfer[3],0,S15C.Read_Data.MDC_Lower_Limit,0,8)BTD(Port_Data.Data_Transfer[4],0,S15C.Read_Data.MDC_Upper_Limit,24,8)BTD(Port_Data.Data_Transfer[5],0,S15C.Read_Data.MDC_Upper_Limit,16,8)BTD(Port_Data.Data_Transfer[6],0,S15C.Read_Data.MDC_Upper_Limit,8,8)BTD(Port_Data.Data_Transfer[7],0,S15C.Read_Data.MDC_Upper_Limit,0,8)BTD(Port_Data.Data_Transfer[8],0,S15C.Read_Data.MDC_Unit,8,8)BTD(Port_Data.Data_Transfer[9],0,S15C.Read_Data.MDC_Unit,0,8)BTD(Port_Data.Data_Transfer[10],0,S15C.Read_Data.MDC_Scale,0,8)OTU(Port_Data.Port_Read.[Port])OTL(Local_Control.6);
   52: NOP();
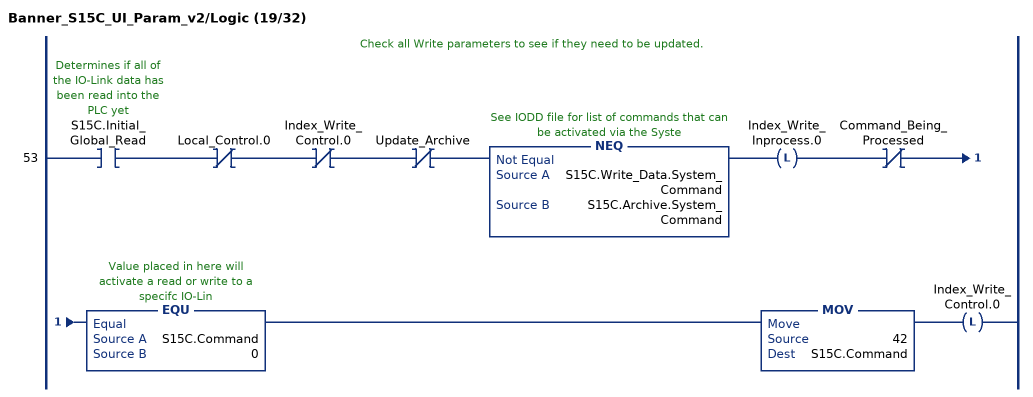
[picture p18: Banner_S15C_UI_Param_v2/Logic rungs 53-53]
   // Check all Write parameters to see if they need to be updated.
   53: XIC(S15C.Initial_Global_Read)XIO(Local_Control.0)XIO(Index_Write_Control.0)XIO(Update_Archive)NEQ(S15C.Write_Data.System_Command,S15C.Archive.System_Command)OTL(Index_Write_Inprocess.0)XIO(Command_Being_Processed)EQU(S15C.Command,0)MOV(42,S15C.Command)OTL(Index_Write_Control.0);
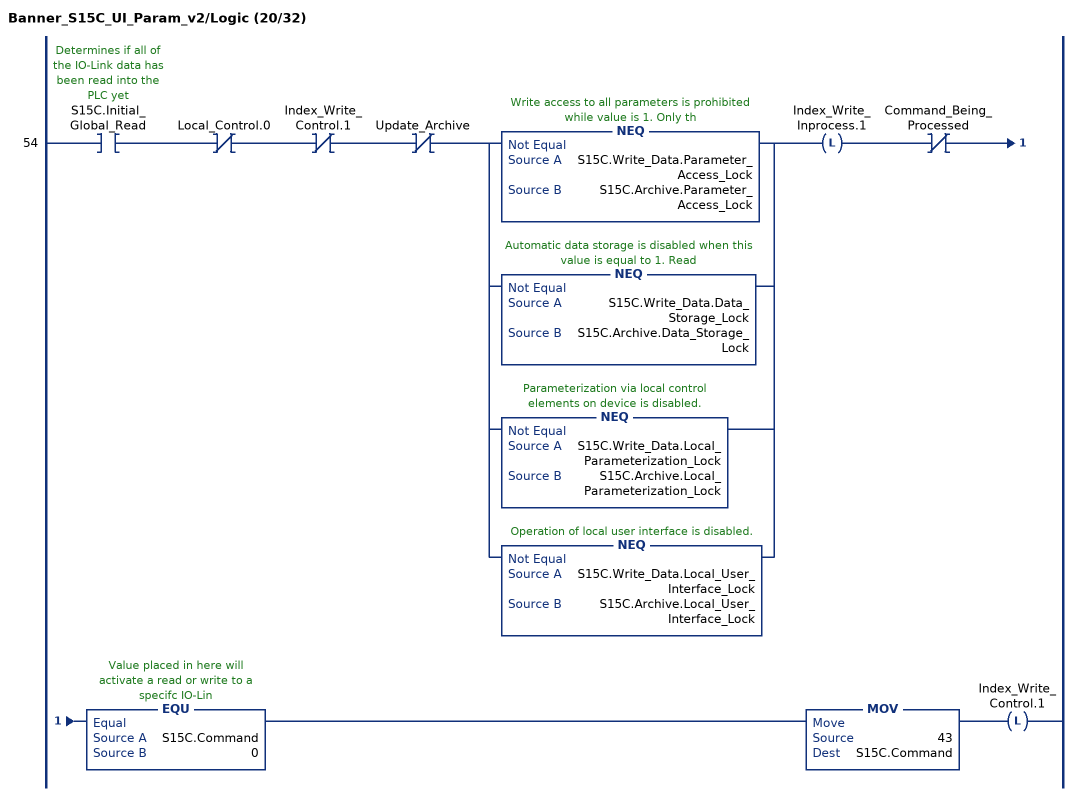
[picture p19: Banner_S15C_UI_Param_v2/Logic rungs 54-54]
   54: XIC(S15C.Initial_Global_Read)XIO(Local_Control.0)XIO(Index_Write_Control.1)XIO(Update_Archive)[NEQ(S15C.Write_Data.Parameter_Access_Lock,S15C.Archive.Parameter_Access_Lock) ,NEQ(S15C.Write_Data.Data_Storage_Lock,S15C.Archive.Data_Storage_Lock) ,NEQ(S15C.Write_Data.Local_Parameterization_Lock,S15C.Archive.Local_Parameterization_Lock) ,NEQ(S15C.Write_Data.Local_User_Interface_Lock,S15C.Archive.Local_User_Interface_Lock) ]OTL(Index_Write_Inprocess.1)XIO(Command_Being_Processed)EQU(S15C.Command,0)MOV(43,S15C.Command)OTL(Index_Write_Control.1);
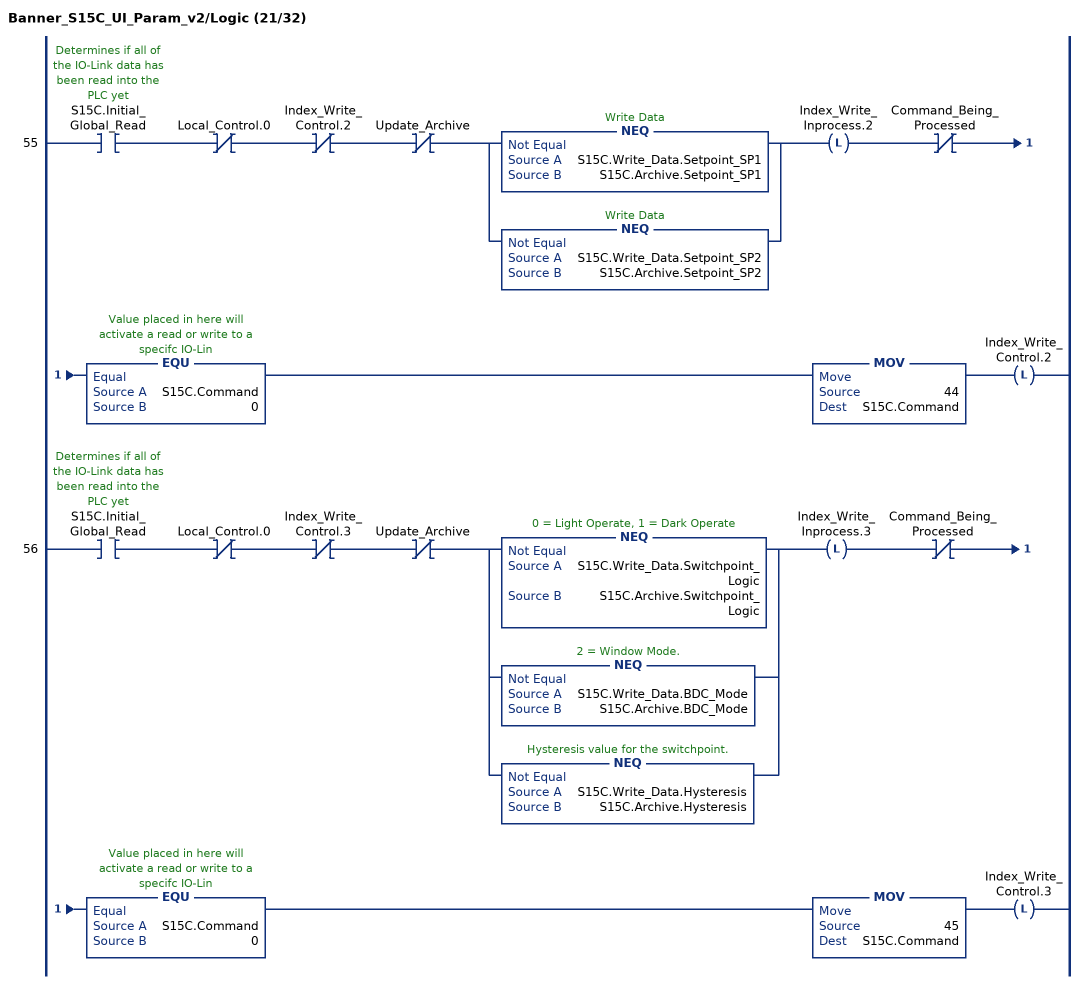
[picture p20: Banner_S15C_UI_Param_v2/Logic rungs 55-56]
   55: XIC(S15C.Initial_Global_Read)XIO(Local_Control.0)XIO(Index_Write_Control.2)XIO(Update_Archive)[NEQ(S15C.Write_Data.Setpoint_SP1,S15C.Archive.Setpoint_SP1) ,NEQ(S15C.Write_Data.Setpoint_SP2,S15C.Archive.Setpoint_SP2) ]OTL(Index_Write_Inprocess.2)XIO(Command_Being_Processed)EQU(S15C.Command,0)MOV(44,S15C.Command)OTL(Index_Write_Control.2);
   56: XIC(S15C.Initial_Global_Read)XIO(Local_Control.0)XIO(Index_Write_Control.3)XIO(Update_Archive)[NEQ(S15C.Write_Data.Switchpoint_Logic,S15C.Archive.Switchpoint_Logic) ,NEQ(S15C.Write_Data.BDC_Mode,S15C.Archive.BDC_Mode) ,NEQ(S15C.Write_Data.Hysteresis,S15C.Archive.Hysteresis) ]OTL(Index_Write_Inprocess.3)XIO(Command_Being_Processed)EQU(S15C.Command,0)MOV(45,S15C.Command)OTL(Index_Write_Control.3);
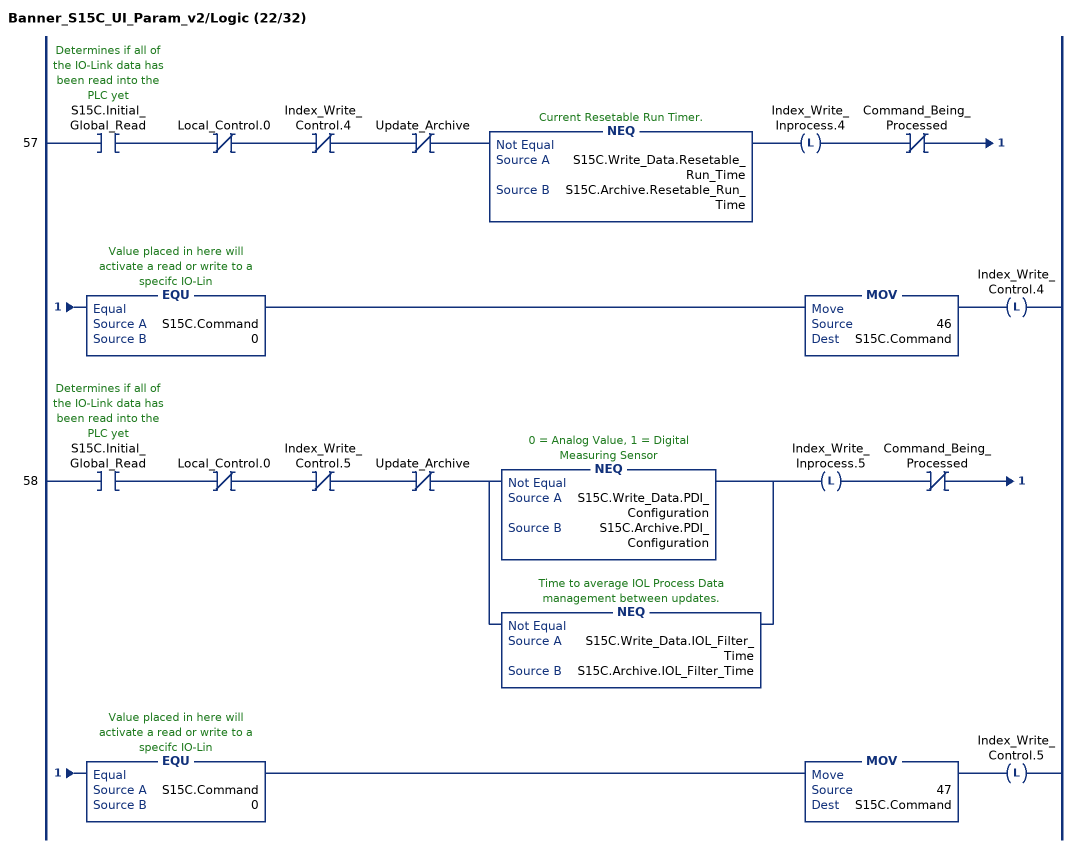
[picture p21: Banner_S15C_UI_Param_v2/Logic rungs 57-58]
   57: XIC(S15C.Initial_Global_Read)XIO(Local_Control.0)XIO(Index_Write_Control.4)XIO(Update_Archive)NEQ(S15C.Write_Data.Resetable_Run_Time,S15C.Archive.Resetable_Run_Time)OTL(Index_Write_Inprocess.4)XIO(Command_Being_Processed)EQU(S15C.Command,0)MOV(46,S15C.Command)OTL(Index_Write_Control.4);
   58: XIC(S15C.Initial_Global_Read)XIO(Local_Control.0)XIO(Index_Write_Control.5)XIO(Update_Archive)[NEQ(S15C.Write_Data.PDI_Configuration,S15C.Archive.PDI_Configuration) ,NEQ(S15C.Write_Data.IOL_Filter_Time,S15C.Archive.IOL_Filter_Time) ]OTL(Index_Write_Inprocess.5)XIO(Command_Being_Processed)EQU(S15C.Command,0)MOV(47,S15C.Command)OTL(Index_Write_Control.5);
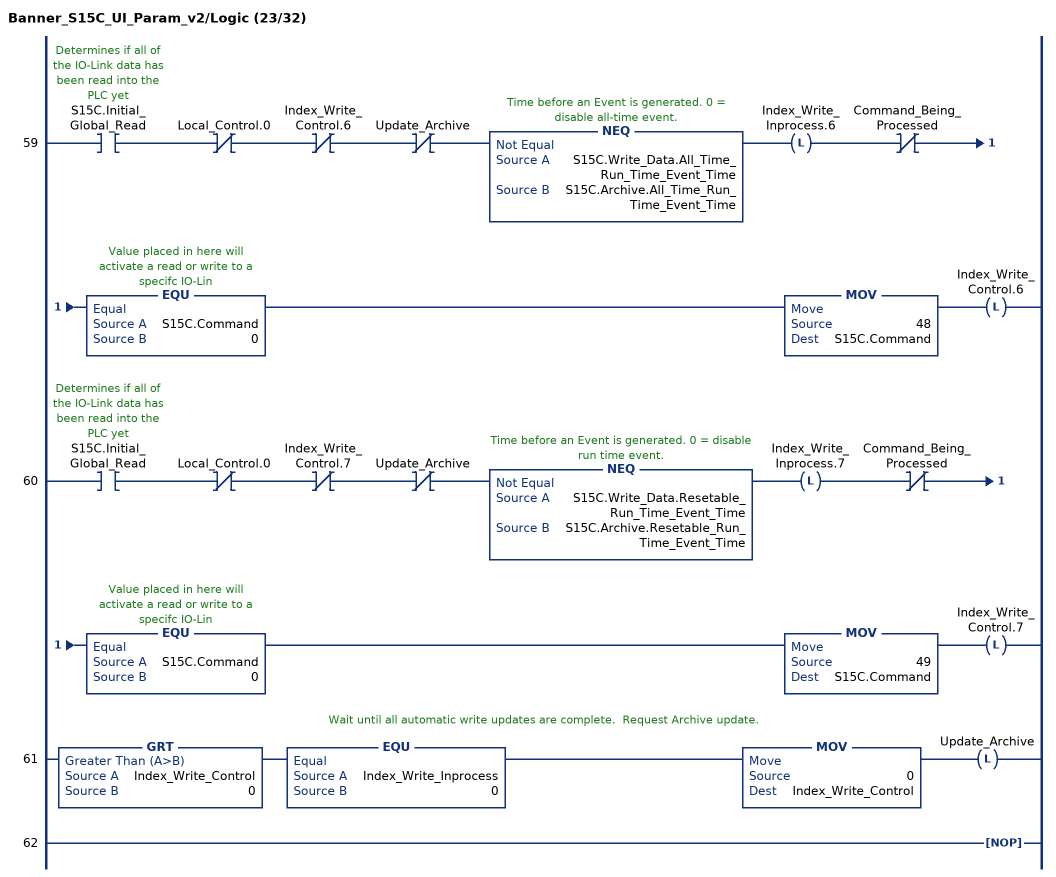
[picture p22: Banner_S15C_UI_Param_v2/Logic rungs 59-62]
   59: XIC(S15C.Initial_Global_Read)XIO(Local_Control.0)XIO(Index_Write_Control.6)XIO(Update_Archive)NEQ(S15C.Write_Data.All_Time_Run_Time_Event_Time,S15C.Archive.All_Time_Run_Time_Event_Time)OTL(Index_Write_Inprocess.6)XIO(Command_Being_Processed)EQU(S15C.Command,0)MOV(48,S15C.Command)OTL(Index_Write_Control.6);
   60: XIC(S15C.Initial_Global_Read)XIO(Local_Control.0)XIO(Index_Write_Control.7)XIO(Update_Archive)NEQ(S15C.Write_Data.Resetable_Run_Time_Event_Time,S15C.Archive.Resetable_Run_Time_Event_Time)OTL(Index_Write_Inprocess.7)XIO(Command_Being_Processed)EQU(S15C.Command,0)MOV(49,S15C.Command)OTL(Index_Write_Control.7);
   // Wait until all automatic write updates are complete.  Request Archive update.
   61: GRT(Index_Write_Control,0)EQU(Index_Write_Inprocess,0)MOV(0,Index_Write_Control)OTL(Update_Archive);
   62: NOP();
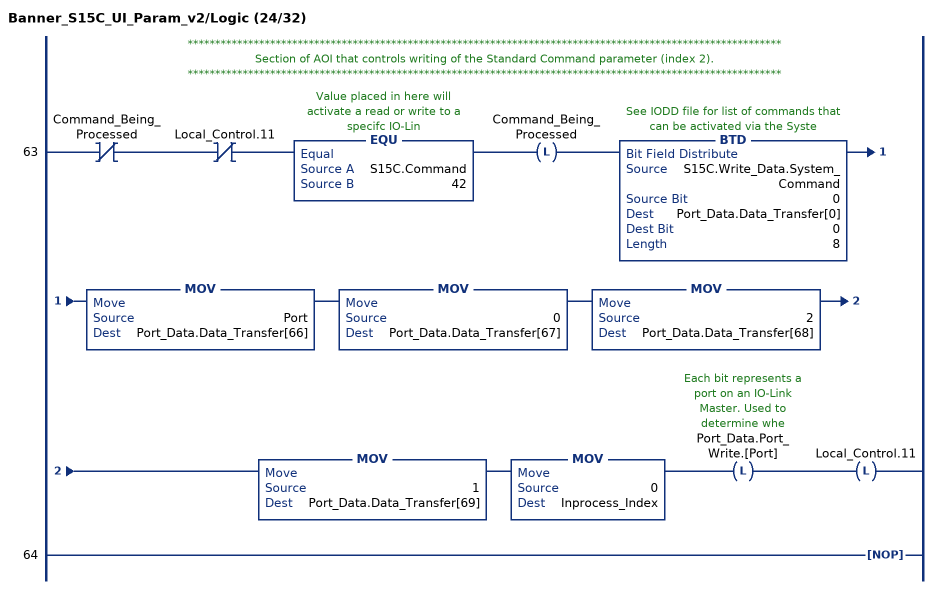
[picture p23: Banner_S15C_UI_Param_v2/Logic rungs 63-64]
   // ************************************************************************************************************
   // Section of AOI that controls writing of the Standard Command parameter (index 2).
   // ************************************************************************************************************
   63: XIO(Command_Being_Processed)XIO(Local_Control.11)EQU(S15C.Command,42)OTL(Command_Being_Processed)BTD(S15C.Write_Data.System_Command,0,Port_Data.Data_Transfer[0],0,8)MOV(Port,Port_Data.Data_Transfer[66])MOV(0,Port_Data.Data_Transfer[67])MOV(2,Port_Data.Data_Transfer[68])MOV(1,Port_Data.Data_Transfer[69])MOV(0,Inprocess_Index)OTL(Port_Data.Port_Write.[Port])OTL(Local_Control.11);
   64: NOP();
